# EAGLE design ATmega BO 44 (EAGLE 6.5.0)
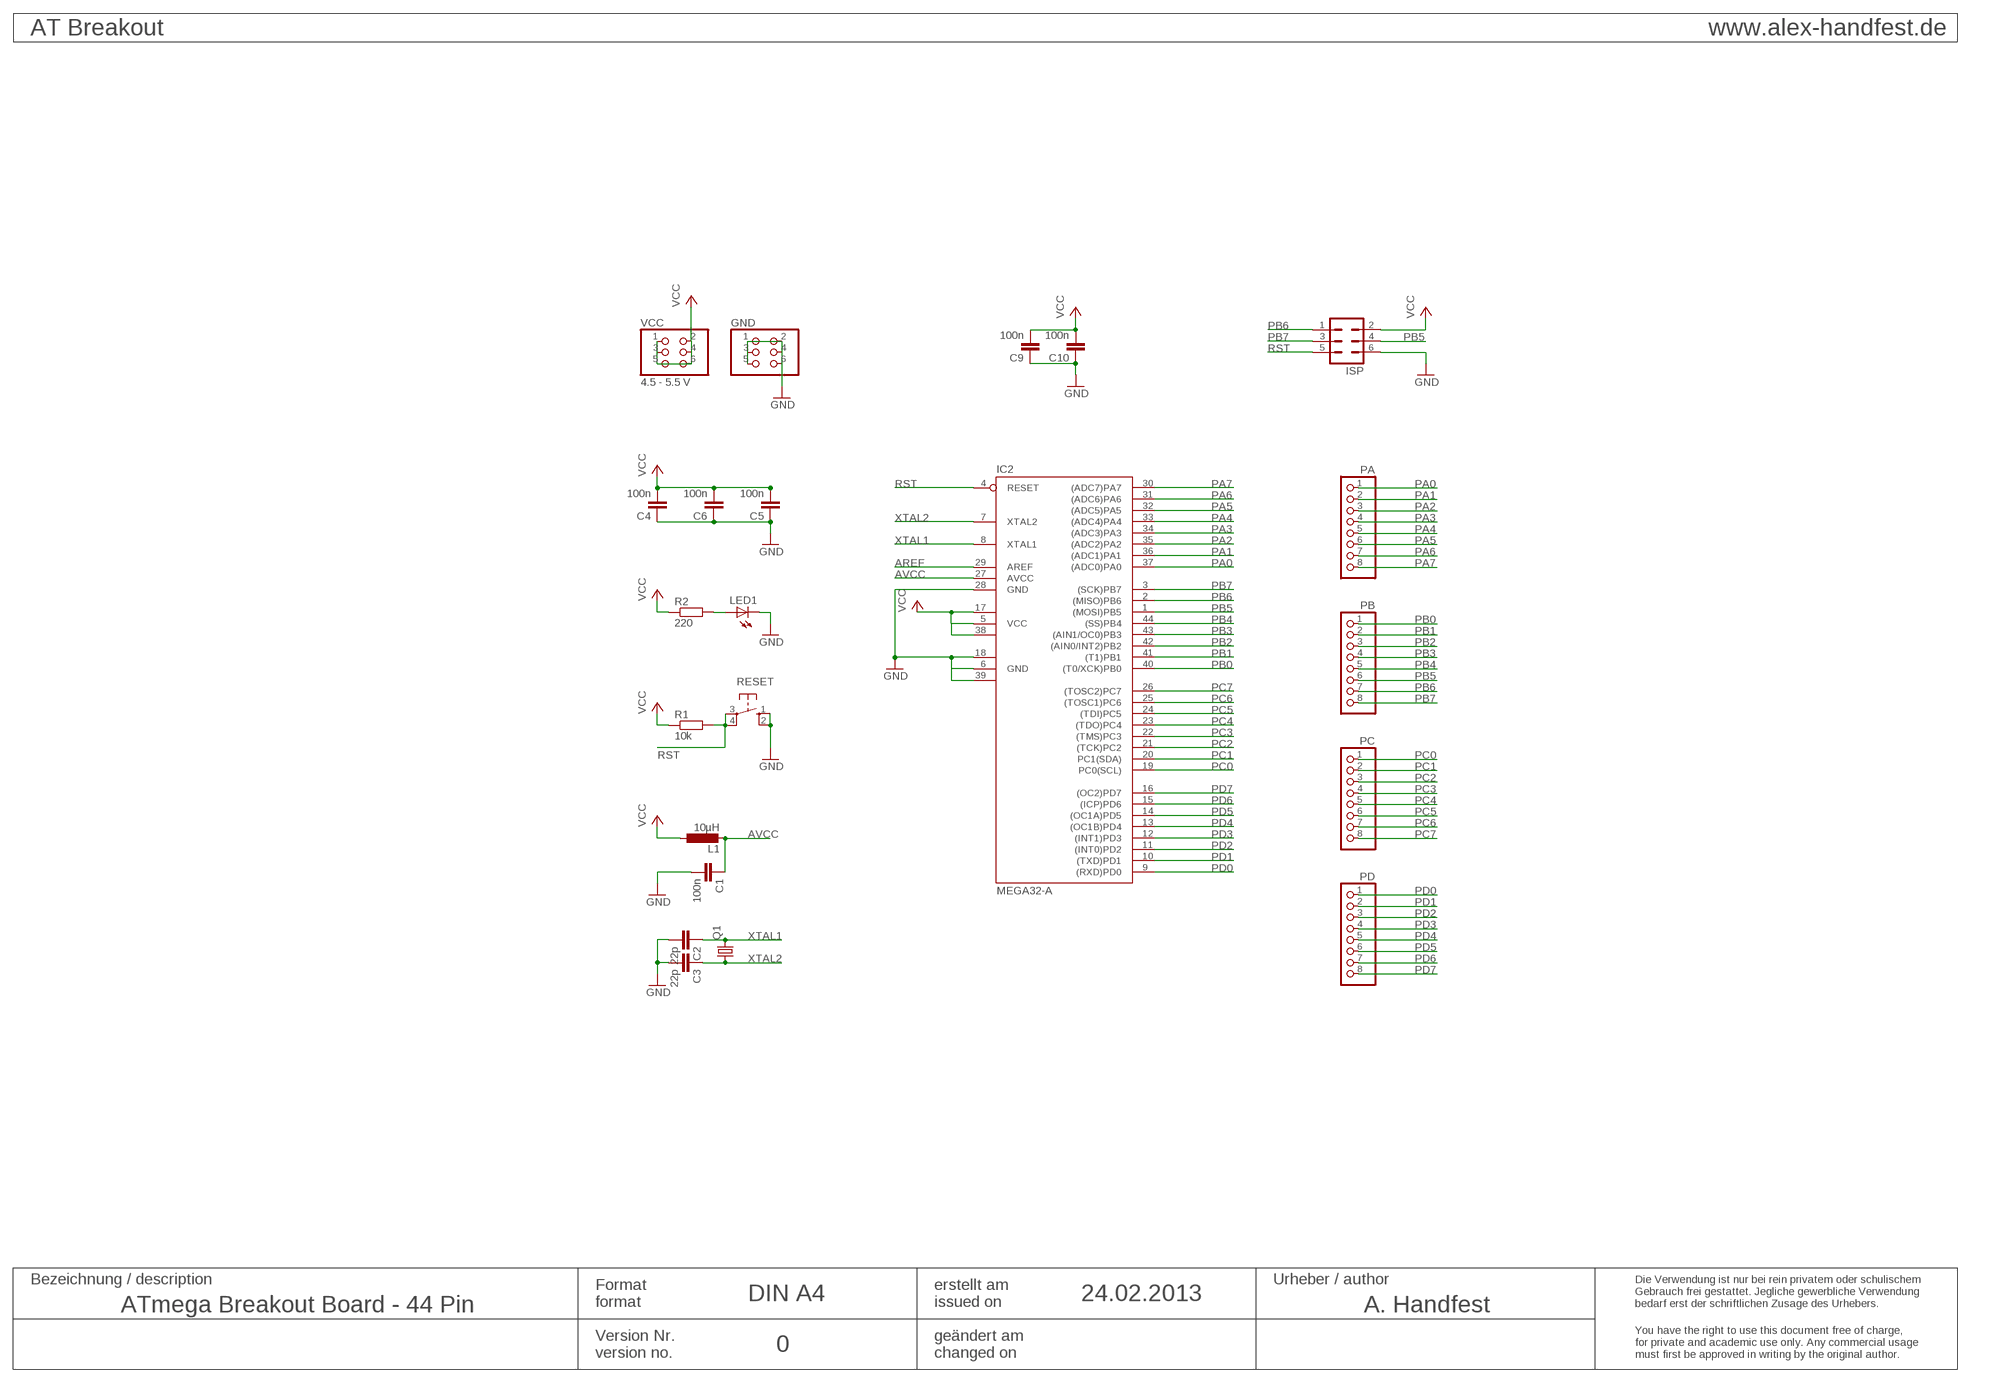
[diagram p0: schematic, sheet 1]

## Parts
C1  100n  C-EUC0805  [C0805]
C2  22p  C-EUC0805  [C0805]
C3  22p  C-EUC0805  [C0805]
C4  100n  C-EUC0805  [C0805]
C5  100n  C-EUC0805  [C0805]
C6  100n  C-EUC0805  [C0805]
C9  100n  C-EUC0805  [C0805]
C10  100n  C-EUC0805  [C0805]
GND  PINHD-2X3  [2X03]
IC2  MEGA32-A  [TQFP44]
ISP  ML6  [ML6]
L1  10µH  L-EUL2012C  [L2012C]
LED1  LEDCHIP-LED0805  [CHIP-LED0805]
PA  PINHD-1X8  [1X08]
PB  PINHD-1X8  [1X08]
PC  PINHD-1X8  [1X08]
PD  PINHD-1X8  [1X08]
Q1  CRYSTALCTS406  [CTS406]
R1  10k  R-EU_R0805  [R0805]
R2  220  R-EU_R0805  [R0805]
RESET  10-XX  [B3F-10XX]
VCC  4.5 - 5.5 V  PINHD-2X3  [2X03]

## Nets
AREF: IC2.29(AREF)
AVCC: C1.1 IC2.27(AVCC) L1.2
GND: C1.2 C2.2 C3.2 C4.1 C5.1 C6.1 C9.1 C10.1 GND.1 GND.2 GND.3 GND.4 GND.5 GND.6 IC2.6(GND) IC2.18(GND1) IC2.28(GND) IC2.39(GND2) ISP.6 LED1.C RESET.1(S) RESET.2(S1)
N$6: LED1.A R2.2
PA0: IC2.37((ADC0)PA0) PA.1
PA1: IC2.36((ADC1)PA1) PA.2
PA2: IC2.35((ADC2)PA2) PA.3
PA3: IC2.34((ADC3)PA3) PA.4
PA4: IC2.33((ADC4)PA4) PA.5
PA5: IC2.32((ADC5)PA5) PA.6
PA6: IC2.31((ADC6)PA6) PA.7
PA7: IC2.30((ADC7)PA7) PA.8
PB0: IC2.40((T0/XCK)PB0) PB.1
PB1: IC2.41((T1)PB1) PB.2
PB2: IC2.42((AIN0/INT2)PB2) PB.3
PB3: IC2.43((AIN1/OC0)PB3) PB.4
PB4: IC2.44((SS)PB4) PB.5
PB5: IC2.1((MOSI)PB5) ISP.4 PB.6
PB6: IC2.2((MISO)PB6) ISP.1 PB.7
PB7: IC2.3((SCK)PB7) ISP.3 PB.8
PC0: IC2.19(PC0(SCL)) PC.1
PC1: IC2.20(PC1(SDA)) PC.2
PC2: IC2.21((TCK)PC2) PC.3
PC3: IC2.22((TMS)PC3) PC.4
PC4: IC2.23((TDO)PC4) PC.5
PC5: IC2.24((TDI)PC5) PC.6
PC6: IC2.25((TOSC1)PC6) PC.7
PC7: IC2.26((TOSC2)PC7) PC.8
PD0: IC2.9((RXD)PD0) PD.1
PD1: IC2.10((TXD)PD1) PD.2
PD2: IC2.11((INT0)PD2) PD.3
PD3: IC2.12((INT1)PD3) PD.4
PD4: IC2.13((OC1B)PD4) PD.5
PD5: IC2.14((OC1A)PD5) PD.6
PD6: IC2.15((ICP)PD6) PD.7
PD7: IC2.16((OC2)PD7) PD.8
RST: IC2.4(RESET) ISP.5 R1.2 RESET.3(P) RESET.4(P1)
VCC: C4.2 C5.2 C6.2 C9.2 C10.2 IC2.5(VCC) IC2.17(VCC1) IC2.38(VCC2) ISP.2 L1.1 R1.1 R2.1 VCC.1 VCC.2 VCC.3 VCC.4 VCC.5 VCC.6
XTAL1: C2.1 IC2.8(XTAL1) Q1.3
XTAL2: C3.1 IC2.7(XTAL2) Q1.1

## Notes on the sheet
- AT Breakout | www.alex-handfest.de
- Bezeichnung / description | Urheber / author
- Format | erstellt am
- DIN A4 | 24.02.2013
- format | issued on
- Die Verwendung ist nur bei rein privatem oder schulischem
  Gebrauch frei gestattet. Jegliche gewerbliche Verwendung 
  bedarf erst der schriftlichen Zusage des Urhebers.
- ATmega Breakout Board - 44 Pin | A. Handfest
- Version Nr. | geändert am
- 0
- version no. | changed on
- You have the right to use this document free of charge,
  for private and academic use only. Any commercial usage
  must first be approved in writing by the original author.

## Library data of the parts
C1-C6 C9 C10 = rcl:C-EU: CAPACITOR, European symbol
GND VCC = pinhead:PINHD-2X3: PIN HEADER
IC2 = atmel:MEGA32: MICROCONTROLLER 32 Kbytes FLASH 2 Kbytes SRAM 1 Kbytes EEPROM USART 8-channel 10 bit ADC Source: www.atmel.com .. doc2503.pdf
ISP = con-harting-ml:ML6: HARTING
L1 = rcl:L-EU: INDUCTOR, European symbol
LED1 = led:LED: LED
PA PB PC PD = pinhead:PINHD-1X8: PIN HEADER
Q1 = crystal:CRYSTAL: CRYSTAL; OC_FARNELL: unknown; OC_NEWARK: unknown
R1 R2 = rcl:R-EU_: RESISTOR, European symbol
RESET = switch-omron:10-XX: OMRON SWITCH

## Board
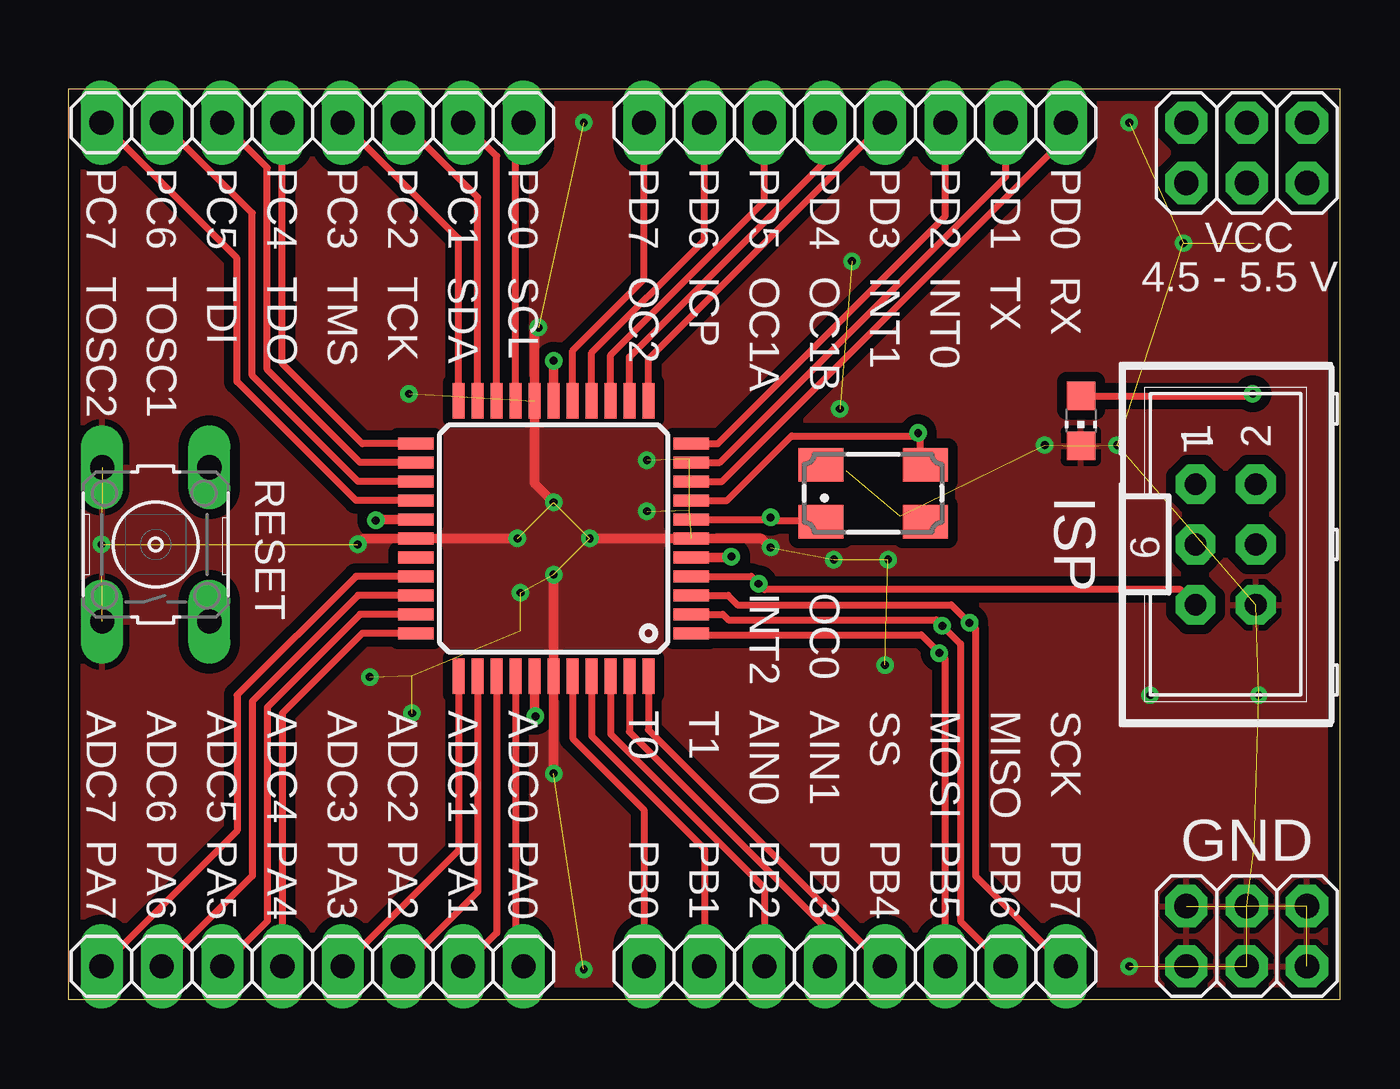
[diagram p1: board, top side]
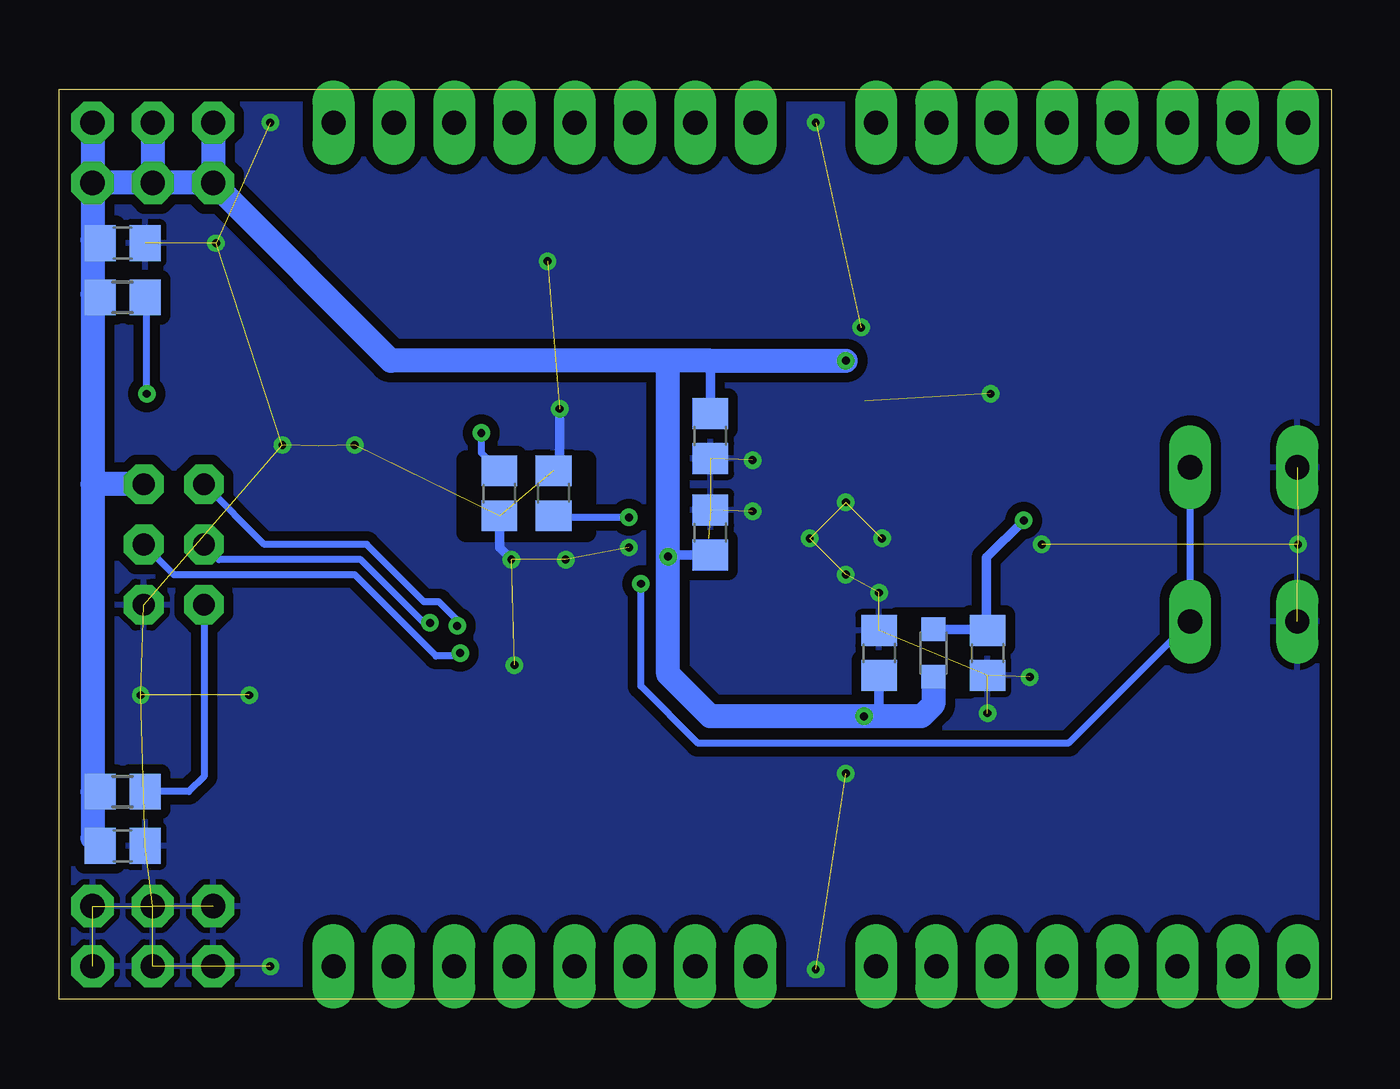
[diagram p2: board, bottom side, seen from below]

Size 53.59 x 38.35 mm. Coordinates in mm from the lower left corner, seen from the top.
Outline: 0,0 53.59,0 53.59,38.35 0,38.35 0,0
Copper layers (1*16): Top 0.035mm / dielectric 1.5mm / Bottom 0.035mm
Design rules "default *": minimum track width 10mil, minimum drill 24mil, track to track 8mil, track to pad 8mil, pad to pad 8mil, via to via 8mil, smd to smd 8mil, copper to edge 20mil, drill to drill 8mil, minimum pad ring 15mil, minimum via ring 8mil, stop-mask expansion 4mil, vias tented up to drill 20mil, thermal gap 10mil
tRestrict: area 31.7,19.6 to 37,22.6
bRestrict: area 31.4,19.7 to 36.4,22.7; area 15.2,13.1 to 18.3,16.1

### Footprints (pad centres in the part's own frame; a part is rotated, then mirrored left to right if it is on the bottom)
C0805 = smd 1.3 x 1.5: 1 -0.95,0; 2 0.95,0
2X03 = drill 1.016 octagon: 1 -2.54,-1.27; 2 -2.54,1.27; 3 0,-1.27; 4 0,1.27; 5 2.54,-1.27; 6 2.54,1.27
TQFP44 = smd 1.5 x 0.5: 1 -5.8,4; 2 -5.8,3.2; 3 -5.8,2.4; 4 -5.8,1.6; 5 -5.8,0.8; 6 -5.8,0; 7 -5.8,-0.8; 8 -5.8,-1.6; 9 -5.8,-2.4; 10 -5.8,-3.2; 11 -5.8,-4; 23 5.8,-4; 24 5.8,-3.2; 25 5.8,-2.4; 26 5.8,-1.6; 27 5.8,-0.8; 28 5.8,0; 29 5.8,0.8; 30 5.8,1.6; 31 5.8,2.4; 32 5.8,3.2; 33 5.8,4 | smd 0.5 x 1.5: 12 -4,-5.8; 13 -3.2,-5.8; 14 -2.4,-5.8; 15 -1.6,-5.8; 16 -0.8,-5.8; 17 0,-5.8; 18 0.8,-5.8; 19 1.6,-5.8; 20 2.4,-5.8; 21 3.2,-5.8; 22 4,-5.8; 34 4,5.8; 35 3.2,5.8; 36 2.4,5.8; 37 1.6,5.8; 38 0.8,5.8; 39 0,5.8; 40 -0.8,5.8; 41 -1.6,5.8; 42 -2.4,5.8; 43 -3.2,5.8; 44 -4,5.8
ML6 = drill 0.914 octagon: 1 -2.54,-1.27; 2 -2.54,1.27; 3 0,-1.27; 4 0,1.27; 5 2.54,-1.27; 6 2.54,1.27
L2012C = smd 1 x 1: 1 -1,0; 2 1,0
CHIP-LED0805 = smd 1.2 x 1.2: A 0,-1.05; C 0,1.05
1X08 = drill 1.016 long: 1 -8.89,0; 2 -6.35,0; 3 -3.81,0; 4 -1.27,0; 5 1.27,0; 6 3.81,0; 7 6.35,0; 8 8.89,0
CTS406 = smd 1.9 x 1.4: 1 -2.2,-1.2; 2 2.2,-1.2; 3 2.2,1.2; 4 -2.2,1.2
R0805 = smd 1.3 x 1.5: 1 -0.95,0; 2 0.95,0
B3F-10XX = drill 1.016 long: 1 -3.251,2.261; 2 3.251,2.261; 3 -3.251,-2.261; 4 3.251,-2.261

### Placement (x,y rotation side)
C1  14.48,14.61 270 bottom
C2  35.05,21.34 270 bottom
C3  32.77,21.34 90 bottom
C4  26.16,19.68 270 bottom
C5  26.16,23.75 90 bottom
C6  19.05,14.61 270 bottom
C9  50.93,6.48 180 bottom
C10  50.93,31.88 180 bottom
GND  49.66,2.67 0 top
IC2  20.45,19.43 180 top
ISP  48.77,19.18 270 top
L1  16.76,14.61 90 bottom
LED1  42.67,24.38 180 top
PA  10.29,1.4 180 top
PB  33.15,1.4 0 top
PC  10.29,36.96 180 top
PD  33.15,36.96 180 top
Q1  33.91,21.34 0 top
R1  50.93,8.76 0 bottom
R2  50.93,29.59 0 bottom
RESET  3.68,19.18 90 top
VCC  49.66,35.69 0 top

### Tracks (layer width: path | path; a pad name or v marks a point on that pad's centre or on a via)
AVCC  (via drill 0.33)
  Top 0.406: IC2.27 12.99,20.23 v12.95,20.19
  Bottom 0.406: L1.2 14.53,15.61 | 14.53,15.61 C1.1 | 14.53,15.61 14.53,18.62 v12.95,20.19
GND  (via drill 0.33)  (40 unrouted)
  Top 0.406: v19.81,28.32 19.65,28.16 IC2.18 19.65,21.75 v20.45,20.95 | v29.59,19.05 29.21,19.43 IC2.6 v21.97,19.43 | v20.45,9.53 IC2.39 v20.45,17.91 | v12.19,19.18 12.45,19.43 IC2.28 v18.92,19.43
  Bottom 0.406: v32.51,24.89 32.51,22.54 C3.2 | C2.2 35.05,19.05 v34.54,18.54
  other vias: 21.72,36.96 21.72,1.27 44.7,1.4 44.7,36.96 46.99,31.88 50.16,12.83 45.59,12.83 1.4,19.18 19.05,17.14 24.38,20.57 24.38,22.73 14.48,12.06 12.7,13.59 32.26,18.54 44.2,23.37 41.15,23.37 14.35,25.53 34.42,14.1 33.02,31.11
  pour Top (isolate 0.406): -0.25,38.61 53.85,38.61 53.85,-0.25 -0.25,-0.25
  pour Bottom (isolate 0.406): -0.25,38.61 53.85,38.61 53.85,-0.25 -0.25,-0.25
N$6  (via drill 0.33)
  Top 0.305: LED1.A 49.82,25.43 v49.91,25.53
  Bottom 0.305: v49.91,25.53 49.91,29.52 R2.2
PA0
  Top 0.305: IC2.37 18.85,1.73 PA.1
PA1
  Top 0.305: IC2.36 18.05,2.81 PA.2
PA2
  Top 0.305: IC2.35 17.25,4.55 PA.3
PA3
  Top 0.305: IC2.34 16.45,6.29 PA.4
PA4
  Top 0.305: IC2.33 12.38,15.43 9.02,12.06 PA.5
PA5
  Top 0.305: IC2.32 12.29,16.23 8.38,12.32 8.38,3.3 PA.6
PA6
  Top 0.305: IC2.31 12.21,17.03 7.75,12.57 7.75,5.21 PA.7
PA7
  Top 0.305: IC2.30 12.12,17.83 7.11,12.83 7.11,7.11 PA.8
PB0
  Top 0.305: IC2.40 21.25,11.01 24.26,8 PB.1
PB1
  Top 0.305: IC2.41 22.05,11.1 26.8,6.35 PB.2
PB2
  Top 0.305: IC2.42 22.85,11.19 29.34,4.7 PB.3
PB3
  Top 0.305: IC2.43 23.65,11.28 31.88,3.05 PB.4
PB4
  Top 0.305: IC2.44 24.45,11.37 PB.5
PB5  (via drill 0.33)
  Top 0.305: IC2.1 26.73,15.43 26.8,15.37 35.94,15.37 v36.7,14.61 36.96,14.35 PB.6
  Bottom 0.305: v36.7,14.61 36.83,14.48 37.72,14.48 41.15,17.91 48.77,17.91 ISP.4
PB6  (via drill 0.33)
  Top 0.305: IC2.2 27.58,16.23 27.81,16 36.58,16 v36.83,15.75 37.59,14.99 37.59,3.3 PB.7
  Bottom 0.305: v36.83,15.75 36.83,16 37.59,16.76 38.23,16.76 40.64,19.18 44.96,19.18 ISP.1
PB7  (via drill 0.33)
  Top 0.305: IC2.3 27.8,17.03 28.19,16.64 37.21,16.64 v37.97,15.88 38.23,15.62 38.23,5.21 PB.8
  Bottom 0.305: v37.97,15.88 38.23,15.88 40.89,18.54 46.86,18.54 ISP.3
PC0
  Top 0.305: IC2.19 18.85,36.63 PC.1
PC1
  Top 0.305: IC2.20 18.05,35.55 PC.2
PC2
  Top 0.305: IC2.21 17.25,33.81 PC.3
PC3
  Top 0.305: IC2.22 16.45,32.07 PC.4
PC4
  Top 0.305: IC2.23 12.38,23.43 9.02,26.8 PC.5
PC5
  Top 0.305: IC2.24 12.29,22.63 8.38,26.54 8.38,35.05 PC.6
PC6
  Top 0.305: IC2.25 12.21,21.83 7.75,26.29 7.75,33.15 PC.7
PC7
  Top 0.305: IC2.26 12.12,21.03 7.11,26.04 7.11,31.24 PC.8
PD0
  Top 0.305: IC2.9 27.55,21.83 42.04,36.32 PD.1
PD1
  Top 0.305: IC2.10 27.46,22.63 39.5,34.67 PD.2
PD2
  Top 0.305: IC2.11 27.37,23.43 36.96,33.02 PD.3
PD3
  Top 0.305: IC2.12 24.45,26.99 PD.4
PD4
  Top 0.305: IC2.13 23.65,27.08 31.88,35.31 PD.5
PD5
  Top 0.305: IC2.14 22.85,27.16 29.34,33.66 PD.6
PD6
  Top 0.305: IC2.15 22.05,27.25 26.8,32 PD.7
PD7
  Top 0.305: IC2.16 21.25,27.34 24.26,30.35 PD.8
RST  (via drill 0.33)
  Top 0.305: IC2.4 28.78,17.83 v29.08,17.53 29.34,17.27 46.86,17.27 ISP.5
  Bottom 0.305: ISP.5 47.5,9.4 48.13,8.76 R1.2 | RESET.4 RESET.3 11.07,10.79 26.67,10.79 29.08,13.21 v29.08,17.53
VCC  (via drill 0.33)
  Top 0.406: IC2.38 19.65,11.98 v19.68,11.94 | IC2.5 27.9,18.63 v27.94,18.67 | IC2.17 v20.45,26.92
  Bottom 0.305: R2.1 52.07,29.59 52.2,29.72 | C10.2 52.07,31.88 52.2,32
  Bottom 0.406: 19.94,12.19 v19.68,11.94 | C4.2 27.87,18.73 v27.94,18.67 | C5.2 26.16,26.92 | R1.1 52.2,8.76 | C6.2 19.05,11.94
  Bottom 1.016: VCC.5 52.2,32 52.2,29.72 52.2,21.72 | 52.2,21.72 52.2,8.76 52.2,6.8 C9.2 | ISP.2 52.2,21.72 | v20.45,26.92 26.16,26.92 28.07,26.92 | L1.1 16.76,12.45 17.27,11.94 19.05,11.94 v19.68,11.94 26.16,11.94 27.94,13.72 v27.94,18.67 27.94,26.8 28.07,26.92 | 28.07,26.92 39.62,26.92 VCC.1 | VCC.1 VCC.3 | VCC.3 VCC.5 | VCC.2 VCC.1 | VCC.4 VCC.3 | VCC.6 VCC.5
XTAL1  (via drill 0.33)
  Top 0.305: IC2.8 27.76,21.03 30.48,23.75 35.69,23.75 v35.81,23.88 35.89,23.8 35.89,22.76 Q1.3
  Bottom 0.305: v35.81,23.88 35.81,23.05 C2.1
XTAL2  (via drill 0.33)
  Top 0.305: IC2.7 29.5,20.23 v29.59,20.32 29.73,20.19 31.71,20.19 Q1.1
  Bottom 0.305: v29.59,20.32 32.06,20.32 C3.1

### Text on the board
tNames: PC7 | PC6 | PC5 | PC4 | PC3 | PC2 | PC1 | PC0 | PD7 | PD6 | PD5 | PD4 | PD3 | PD2 | PD1 | PD0 | TOSC2 | TOSC1 | TDI | TDO | TMS | TCK | SDA | SCL | OC2 | ICP | OC1A | OC1B | INT1 | INT0 | TX | RX | 1 | INT2 | OC0 | ADC7 | ADC6 | ADC5 | ADC4 | ADC3 | ADC2 | ADC1 | ADC0 | T0 | T1 | AIN0 | AIN1 | SS | MOSI | MISO | SCK | PA7 | PA6 | PA5 | PA4 | PA3 | PA2 | PA1 | PA0 | PB0 | PB1 | PB2 | PB3 | PB4 | PB5 | PB6 | PB7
